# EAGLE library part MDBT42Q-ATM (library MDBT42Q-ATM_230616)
Raytac Corporation Part Number: (nRF52832) MDBT42Q-ATM / MDBT42Q-PATM Bluetooth Low Energy Module based on Noridc nRF52832 Size: 16x10mm Source: Raytac datasheet
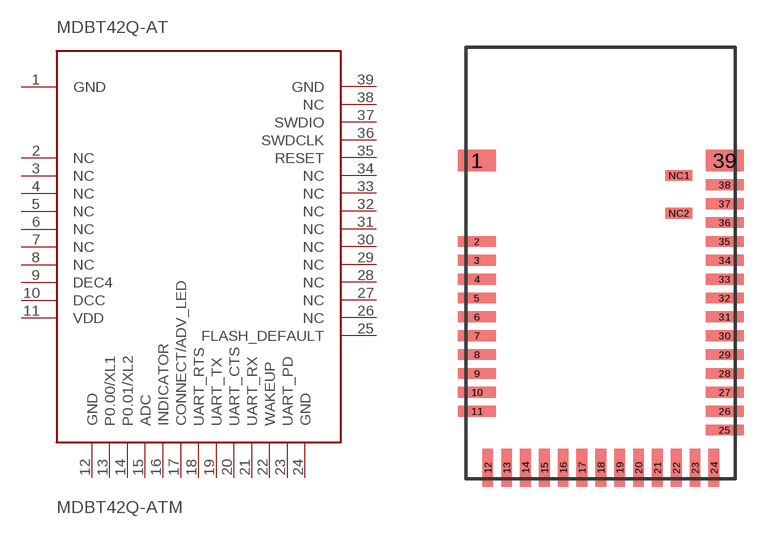
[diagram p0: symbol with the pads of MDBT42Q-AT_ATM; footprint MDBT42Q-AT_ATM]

Designator prefix MDBT42Q-AT

## MDBT42Q-ATM  [MDBT42Q-AT_ATM]
1  GND
2  NC
3  NC
4  NC
5  NC
6  NC
7  NC
8  NC
9  DEC4
10  DCC
11  VDD
12  GND
13  P0.00/XL1
14  P0.01/XL2
15  ADC
16  INDICATOR
17  CONNECT/ADV_LED
18  UART_RTS
19  UART_TX
20  UART_CTS
21  UART_RX
22  WAKEUP
23  UART_PD
24  GND
25  FLASH_DEFAULT
26  NC
27  NC
28  NC
29  NC
30  NC
31  NC
32  NC
33  NC
34  NC
35  RESET
36  SWDCLK
37  SWDIO
38  NC
39  GND

## Footprint MDBT42Q-AT_ATM (pad centres in mm)
Raytac Corporation Part Number: (nRF52832) MDBT42Q-ATM / MDBT42Q-PATM (nRF52810) MDBT42Q-AT / MDBT42Q-PAT (nRF52811) MDBT42Q-ATL / MDBT42Q-PATL Bluetooth Low Energy Module based on Noridc nRF52832 /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
smd 1.4 x 0.8: 1 -4.6,3.8; 39 4.6,3.8
smd 1.4 x 0.4: 2 -4.6,0.8; 3 -4.6,0.1; 4 -4.6,-0.6; 5 -4.6,-1.3; 6 -4.6,-2; 7 -4.6,-2.7; 8 -4.6,-3.4; 9 -4.6,-4.1; 10 -4.6,-4.8; 11 -4.6,-5.5; 25 4.6,-6.2; 26 4.6,-5.5; 27 4.6,-4.8; 28 4.6,-4.1; 29 4.6,-3.4; 30 4.6,-2.7; 31 4.6,-2; 32 4.6,-1.3; 33 4.6,-0.6; 34 4.6,0.1; 35 4.6,0.8; 36 4.6,1.5; 37 4.6,2.2; 38 4.6,2.9
smd 0.4 x 1.4: 12 -4.2,-7.6; 13 -3.5,-7.6; 14 -2.8,-7.6; 15 -2.1,-7.6; 16 -1.4,-7.6; 17 -0.7,-7.6; 18 0,-7.6; 19 0.7,-7.6; 20 1.4,-7.6; 21 2.1,-7.6; 22 2.8,-7.6; 23 3.5,-7.6; 24 4.2,-7.6
smd 1 x 0.4: NC1 2.9,3.25; NC2 2.9,1.85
